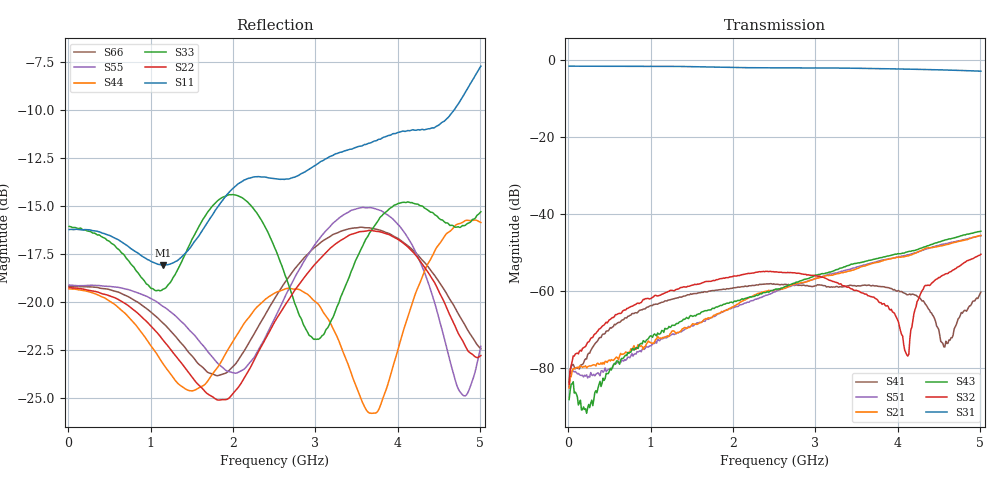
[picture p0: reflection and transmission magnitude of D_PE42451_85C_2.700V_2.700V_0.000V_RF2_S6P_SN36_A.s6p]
! Device ID: PE42451
! Serial: 36
! Insertion: A
! Temp: 85C
! VDD: 2.700
! Control_Hi: 100.000
! Control_Lo: 0.000
! Logic State: RF2
! Port 1: RFC
! Port 2: RF1
! Port 3: RF2
! Port 4: RF3
! Port 5: RF4
! Port 6: RF5
! V1 = 0.00
! V2 = 2.70
! V3 = 0.00
! V4 = 0.00
! IDD: 1.137980e-05
#  Hz  S  RI  R  50
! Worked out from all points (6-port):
!   401 points, 10 MHz to 5.01 GHz, reference 50 ohm
!   strongest paths, dB at 10 MHz, 1.26 GHz, 2.51 GHz, 3.76 GHz, 5.01 GHz:
!     S31: -1.6, -1.7, -2.0, -2.2, -2.9
!     S32: -84.1, -59.8, -55.0, -62.4, -50.4
!     S43: -88.2, -68.8, -59.6, -51.5, -44.5
!     S21: -85.2, -70.3, -59.6, -52.5, -45.6
!     S51: -85.0, -71.2, -60.2, -52.2, -45.6
!     S41: -83.6, -62.1, -58.2, -58.7, -60.2
!   lowest |S11| = -18.1 dB at 1.147 GHz (marker M1), VSWR 1.28, Z = 58.5 - j10.6 ohm
!   |S11| at or under -10 dB: start of sweep to 4.689 GHz
